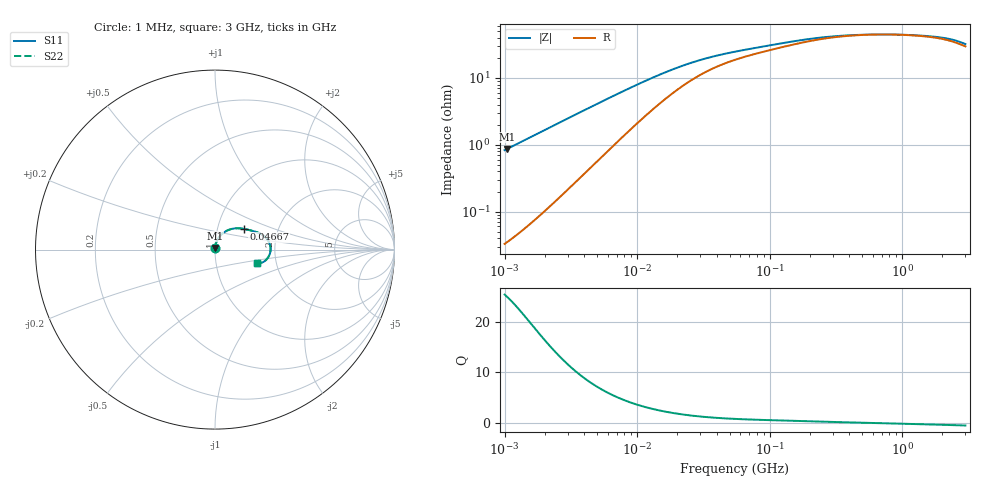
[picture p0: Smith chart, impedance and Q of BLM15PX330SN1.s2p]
! BLM15PX330SN1
# Hz S RI R 50
!Freq.(Hz) S11(Real) S11(Imag) S21(Real) S21(Imag) S12(Real) S12(Imag) S22(Real) S22(Imag)
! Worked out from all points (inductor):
!   401 points, 1 MHz to 3 GHz, reference 50 ohm
!   read as one part in series: L = 132 nH near 1.041 MHz
!   highest Q = 24.9 at 1.041 MHz (marker M1), where L = 132 nH
!   self-resonance near 758.3 MHz
!   S11 on the Smith chart (normalised r, x): 1 MHz: 1.00, +0.02; 46.67 MHz: 1.34, +0.32; 3 GHz: 1.60, -0.25
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1000000  0.000397 0.00831  0.9996 -0.00831  0.9996 -0.00831  0.000397 0.00831
1040844  0.000422 0.00865  0.9996 -0.00865  0.9996 -0.00865  0.000422 0.00865
2139570  0.00145 0.0177  0.9985 -0.0177  0.9985 -0.0177  0.00145 0.0177
3823119  0.00436 0.0312  0.9956 -0.0312  0.9956 -0.0312  0.00436 0.0312
5938264  0.0101 0.0471  0.9899 -0.0471  0.9899 -0.0471  0.0101 0.0471
8345207  0.0189 0.0634  0.9811 -0.0634  0.9811 -0.0634  0.0189 0.0634
1.126754e7  0.0319 0.08  0.9681 -0.08  0.9681 -0.08  0.0319 0.08
1.461624e7  0.0485 0.0947  0.9515 -0.0947  0.9515 -0.0947  0.0485 0.0947
1.934349e7  0.072 0.1081  0.928 -0.1081  0.928 -0.1081  0.072 0.1081
2.559965e7  0.0999 0.1166  0.9001 -0.1166  0.9001 -0.1166  0.0999 0.1166
3.387922e7  0.1288 0.1189  0.8712 -0.1189  0.8712 -0.1189  0.1288 0.1189
4.666789e7  0.1595 0.1158  0.8405 -0.1158  0.8405 -0.1158  0.1595 0.1158
5.477226e7  0.1733 0.113  0.8267 -0.113  0.8267 -0.113  0.1733 0.113
1.219755e8  0.2354 0.0963  0.7646 -0.0963  0.7646 -0.0963  0.2354 0.0963
2.094008e8  0.2741 0.0751  0.7259 -0.0751  0.7259 -0.0751  0.2741 0.0751
2.827291e8  0.2903 0.0586  0.7097 -0.0586  0.7097 -0.0586  0.2903 0.0586
3.894533e8  0.3019 0.0394  0.6981 -0.0394  0.6981 -0.0394  0.3019 0.0394
8.005644e8  0.3096 -0.00314  0.6904 0.00314  0.6904 0.00314  0.3096 -0.00314
1.294266e9  0.3024 -0.0313  0.6976 0.0313  0.6976 0.0313  0.3024 -0.0313
1.893158e9  0.2868 -0.0553  0.7132 0.0553  0.7132 0.0553  0.2868 -0.0553
2.407135e9  0.2667 -0.0703  0.7333 0.0703  0.7333 0.0703  0.2667 -0.0703
3e9  0.2364 -0.0732  0.7636 0.0732  0.7636 0.0732  0.2364 -0.0732
